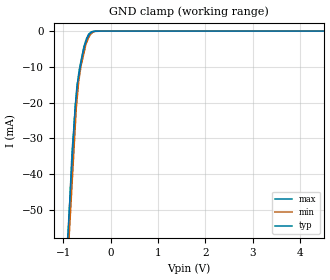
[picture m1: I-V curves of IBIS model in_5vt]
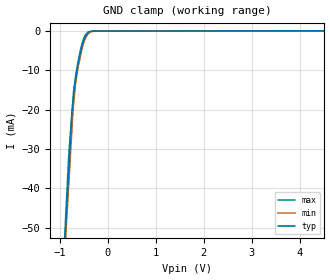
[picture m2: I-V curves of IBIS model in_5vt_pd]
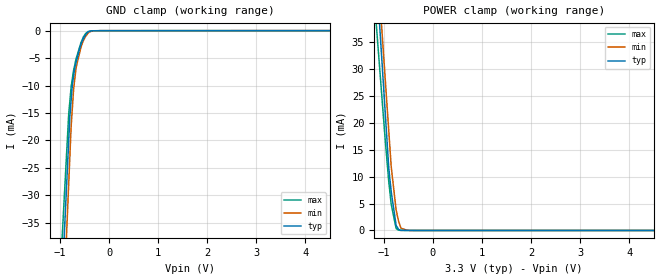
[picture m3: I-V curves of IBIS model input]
|Texas Instruments Incorporated
|112dB SNR Stereo ADC with Differential Inputs
[IBIS Ver]   4.0
[File Name] pcm1804.ibs
[File Rev] 3.0
[Date]   10-06-2009
[Notes]  Quality Check of this IBIS model: Model Passes IBIS Check. Model
   parses into ICX IS. Simulates with Hyperlynx.
   1. MIN TYP MAX information is based on Temperature and Voltage
   characteristics only.
   2. Package information extracted using Tektronix IConnect Software.
[Source]   Texas Instruments Incorporated.
   Analog-eLab, HPA
   12500 TI Blvd
   Dallas, TX -75243
   For Support e-mail: elab_ibis@list.ti.com
[Disclaimer]
| This model is designed as an aid for customers of Texas Instruments.
| TI and its licensors and suppliers make no warranties, either expressed
| or implied, with respect to this  model, including the warranties of
| merchantability or fitness for a particular purpose. The model is
| provided solely on an "as is" basis. The entire risk as to its quality
| and performance is with the customer.
[Copyright]
| (C) Copyright 2011 Texas Instruments Incorporated. All rights reserved.
[Component] PCM1804
[Manufacturer] TI
[Package]
| variable   typ   min   max
R_pkg  1.000E-02   1.000E-02   1.000E-02
L_pkg  2.970E-09   2.790E-09   3.150E-09
C_pkg  4.580E-13   1.880E-13   7.280E-13
[Pin] signal_name  model_name  R_pin  L_pin C_pin
1   VREFL   term   1.000E-02   3.150E-09   7.280E-13
2   AGNDL   GND   1.000E-02   3.090E-09   6.380E-13
3   VCOML   POWER   1.000E-02   3.030E-09   5.480E-13
4   VINL_P   term   1.000E-02   2.970E-09   4.580E-13
5   VINL_M   term   1.000E-02   2.910E-09   3.680E-13
6   FMT0   in_5vt_pd  1.000E-02   2.850E-09   2.780E-13
7   FMT1   in_5vt_pd  1.000E-02   2.790E-09   1.880E-13
8   S/*M   in_5vt_pd  1.000E-02   2.790E-09   1.880E-13
9   OSR0   in_5vt_pd  1.000E-02   2.850E-09   2.780E-13
10  OSR1   in_5vt_pd  1.000E-02   2.910E-09   3.680E-13
11  OSR2   in_5vt_pd  1.000E-02   2.970E-09   4.580E-13
12  BYPAS   input   1.000E-02   3.030E-09   5.480E-13
13  DGND   GND   1.000E-02   3.090E-09   6.380E-13
14  VDD   POWER   1.000E-02   3.150E-09   7.280E-13
15  DATA/DSDR   output   1.000E-02   3.150E-09   7.280E-13
16  BCK/DSDL   bidir   1.000E-02   3.090E-09   6.380E-13
17  LRCK/DSDBCK bidir   1.000E-02   3.030E-09   5.480E-13
18  SCKI   in_5vt   1.000E-02   2.970E-09   4.580E-13
19  *RST   in_5vt_pd  1.000E-02   2.910E-09   3.680E-13
20  OVFR   output   1.000E-02   2.850E-09   2.780E-13
21  OVFL   output   1.000E-02   2.790E-09   1.880E-13
22  VCC   POWER   1.000E-02   2.790E-09   1.880E-13
23  AGND   GND   1.000E-02   2.850E-09   2.780E-13
24  VINR_M   term   1.000E-02   2.910E-09   3.680E-13
25  VINR_P   term   1.000E-02   2.970E-09   4.580E-13
26  VCOMR   POWER   1.000E-02   3.030E-09   5.480E-13
27  AGNDR   GND   1.000E-02   3.090E-09   6.380E-13
28  VREFR   term   1.000E-02   3.150E-09   7.280E-13
[Diff Pin] inv_pin vdiff tdelay_typ tdelay_min tdelay_max
4  5   NA   NA  NA  NA
25 24  NA   NA  NA  NA
[Model]  term
Model_type Terminator
C_comp   0   0   0
[Voltage Range]  5.00  4.75  5.25
[Temperature Range] 25   70   -10
| Models and submodels in the file (6): in_5vt (Input), in_5vt_pd (Input), input (Input), bidir (I/O), output (Output), term (Terminator)
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[Model] in_5vt
Model_type Input
Vinl = 800.000mV
Vinh = 2.00000V
C_comp 768.000fF 764.000fF 773.000fF
| variable typ   min   max
[Voltage Range] 3.30000V 3.00000V 3.60000V
[POWER Clamp Reference] 3.30000V 3.00000V 3.60000V
[GND Clamp Reference] 0.00000V 0.00000V 0.00000V
[Temperature Range] 25   70   -10
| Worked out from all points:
|   GND clamp passes 1 mA (typ) near -0.45 V on its own axis
[GND Clamp]
-3.3V     -616.3mA   -636.6mA   -756.7mA
-815mV    -36.39mA   -42.85mA   -33.79mA
-750mV    -21.22mA   -27.32mA   -22.18mA
-725mV    -17.9mA    -21.34mA   -17.72mA
-700mV    -14.58mA   -17.74mA   -14.44mA
-675mV    -12.65mA   -14.13mA   -11.95mA
-625mV    -8.797mA   -9.733mA   -8.324mA
-550mV    -4.129mA   -5.334mA   -3.734mA
-475mV    -1.51mA    -2.086mA   -1.135mA
-415mV    -442.1uA   -791.5uA   -234.8uA
-162.5mV  -2.763uA   -4.202uA   -2.255uA
6.6V      4.031uA    5.215uA    2.671uA
[POWER Clamp]
-3.3V     0A         0A         0A
6.6V      0A         0A         0A
[Model] in_5vt_pd
Model_type Input
Vinl = 800.000mV
Vinh = 2.00000V
C_comp 1.20000pF 1.19000pF 1.21000pF
| variable typ   min   max
[Voltage Range] 3.30000V 3.00000V 3.60000V
[POWER Clamp Reference] 3.30000V 3.00000V 3.60000V
[GND Clamp Reference] 0.00000V 0.00000V 0.00000V
[Temperature Range] 25   70   -10
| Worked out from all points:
|   GND clamp passes 1 mA (typ) near -0.45 V on its own axis
[GND Clamp]
-3.3V     -590.1mA   -562.6mA   -646.1mA
-815mV    -35.46mA   -39.02mA   -31.39mA
-750mV    -20.95mA   -25.32mA   -21mA
-725mV    -17.72mA   -20.05mA   -17mA
-700mV    -14.5mA    -16.82mA   -13.99mA
-675mV    -12.6mA    -13.59mA   -11.65mA
-625mV    -8.805mA   -9.481mA   -8.172mA
-550mV    -4.184mA   -5.245mA   -3.727mA
-475mV    -1.562mA   -2.081mA   -1.162mA
-415mV    -476.6uA   -799.9uA   -259.5uA
-162.5mV  -13.48uA   -12.24uA   -15.1uA
6.6V      98.52uA    79.62uA    118.4uA
[POWER Clamp]
-3.3V     0A         0A         0A
6.6V      0A         0A         0A
[Model] input
Model_type Input
Vinl = 800.000mV
Vinh = 2.00000V
C_comp 1.57000pF 1.57000pF 1.57000pF
| variable typ   min   max
[Voltage Range] 3.30000V 3.00000V 3.60000V
[POWER Clamp Reference] 3.30000V 3.00000V 3.60000V
[GND Clamp Reference] 0.00000V 0.00000V 0.00000V
[Temperature Range] 25   70   -10
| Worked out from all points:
|   GND clamp passes 1 mA (typ) near -0.50 V on its own axis
|   POWER clamp passes 1 mA (typ) near -0.75 V on its own axis
[GND Clamp]
-3.3V     -489.3mA   -548.8mA   -432mA
-825mV    -20.18mA   -27.99mA   -15.27mA
-800mV    -15.44mA   -22.73mA   -12.75mA
-775mV    -12.65mA   -17.47mA   -10.23mA
-750mV    -9.853mA   -14.08mA   -8.737mA
-725mV    -8.284mA   -10.69mA   -7.241mA
-675mV    -5.835mA   -6.795mA   -5.15mA
-575mV    -2.556mA   -3.008mA   -2.193mA
-500mV    -989.8uA   -1.394mA   -805.7uA
-425mV    -260.2uA   -416.9uA   -136.5uA
-162.5mV  -1.906uA   -2.428uA   -5.301uA
6.6V      4.92uA     15.75uA    6.215uA
[POWER Clamp]
-3.3V     353.4mA    338.3mA    291.3mA
-1.225V   57.9mA     61.82mA    46.61mA
-1.125V   43.66mA    48.49mA    34.81mA
-1.075V   36.54mA    41.83mA    28.91mA
-1.025V   29.42mA    35.16mA    23.02mA
-900mV    11.61mA    18.51mA    9.098mA
-850mV    7.192mA    11.84mA    4.85mA
-750mV    960.8uA    3.808mA    377.6uA
-700mV    185.3uA    1.716mA    59.42uA
-650mV    29.02uA    406.9uA    13.02uA
-475mV    13.4uA     11.01uA    8.09uA
6.6V      0A         0A         0A
